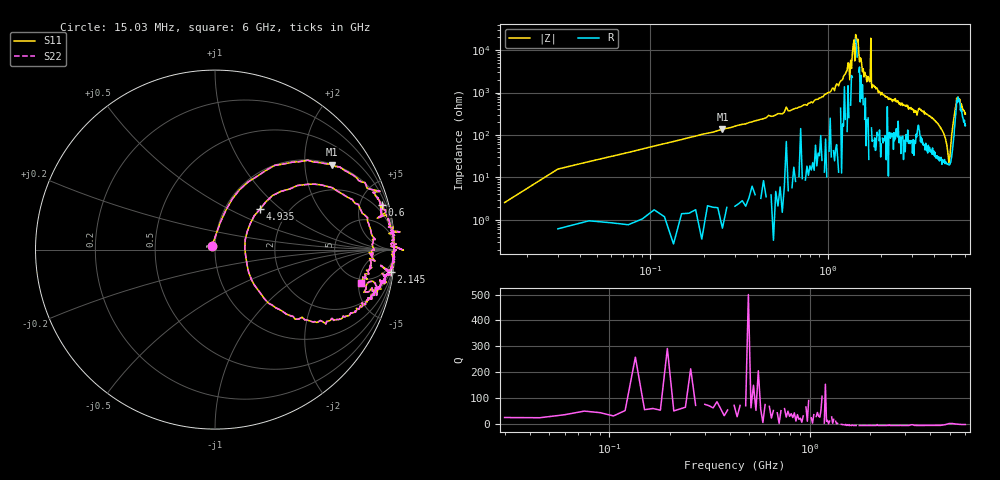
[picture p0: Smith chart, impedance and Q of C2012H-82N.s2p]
!	Network	Analyzer	HP8753E.07.74:	Oct	30	2002	Serial	No.	JP38451487
!	Hewlett-Packard
!	28	Aug	2009	10:29:47
!	Frequency	S11	S21	S12	S22
#	HZ	S	RI	R	50
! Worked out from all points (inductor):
!   400 points, 15.03 MHz to 6 GHz, reference 50 ohm
!   read as one part in series: L = 82.9 nH near 45.03 MHz
!   highest Q = 71.1 at 255 MHz (marker M1), where L = 85.5 nH
!   self-resonance near 1.32 GHz
!   S11 on the Smith chart (normalised r, x): 15.03 MHz: 0.96, +0.03; 600 MHz: 1.09, +7.38; 2.145 GHz: 1, -16; 4.935 GHz: 1.45, +0.75; 6 GHz: 4.35, -5.32
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1.502992e7  -0.0178 0.0181  1.02 -0.0181  1.02 -0.0181  -0.0178 0.0181
6.00297e7  0.0957 0.281  0.904 -0.281  0.904 -0.281  0.0957 0.281
2.550287e8  0.652 0.474  0.348 -0.474  0.348 -0.474  0.652 0.474
6.00027e8  0.929 0.251  0.0714 -0.251  0.0714 -0.251  0.929 0.251
1.020025e9  0.986 0.0967  0.0135 -0.0967  0.0135 -0.0967  0.986 0.0967
1.335023e9  1.05 -0.00348  -0.0526 0.00348  -0.0526 0.00348  1.05 -0.00348
1.410023e9  0.996 0.00433  0.00375 -0.00433  0.00375 -0.00433  0.996 0.00433
1.425023e9  1 0.018  -0.00067 -0.018  -0.00067 -0.018  1 0.018
1.440023e9  0.997 -0.00272  0.0033 0.00272  0.0033 0.00272  0.997 -0.00272
1.665022e9  0.99 -0.0542  0.00986 0.0542  0.00986 0.0542  0.99 -0.0542
1.740021e9  0.995 -0.0537  0.00464 0.0537  0.00464 0.0537  0.995 -0.0537
1.755021e9  1 -0.00519  -0.00085 0.00519  -0.00085 0.00519  1 -0.00519
1.770021e9  0.991 -0.0602  0.00916 0.0602  0.00916 0.0602  0.991 -0.0602
1.785021e9  0.99 -0.0766  0.0102 0.0766  0.0102 0.0766  0.99 -0.0766
2.01002e9  0.983 -0.1  0.0166 0.1  0.0166 0.1  0.983 -0.1
2.145019e9  0.98 -0.125  0.0202 0.125  0.0202 0.125  0.98 -0.125
3.015015e9  0.926 -0.22  0.0739 0.22  0.0739 0.22  0.926 -0.22
4.00501e9  0.802 -0.332  0.198 0.332  0.198 0.332  0.802 -0.332
4.935005e9  0.253 0.228  0.747 -0.228  0.747 -0.228  0.253 0.228
5.010005e9  0.459 0.357  0.541 -0.357  0.541 -0.357  0.459 0.357
5.355003e9  0.893 0.0563  0.107 -0.0563  0.107 -0.0563  0.893 0.0563
6e9  0.812 -0.187  0.188 0.187  0.188 0.187  0.812 -0.187
